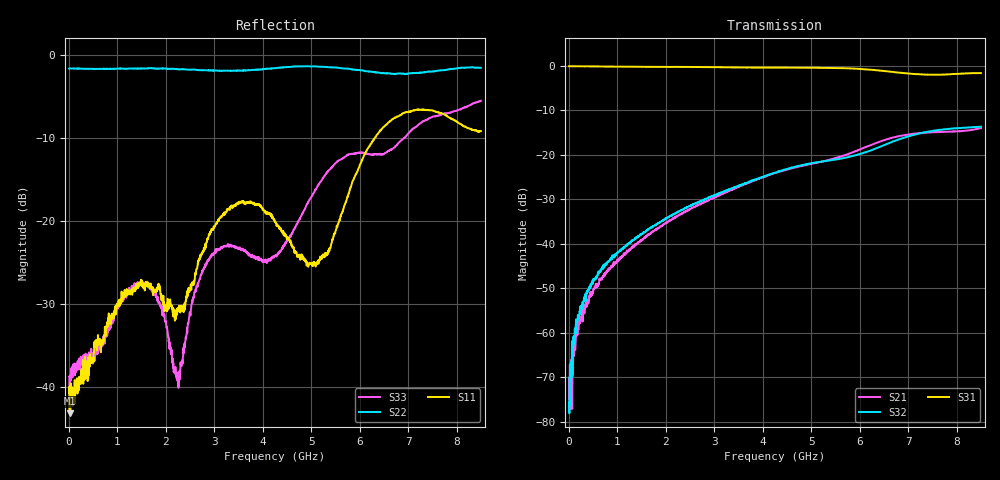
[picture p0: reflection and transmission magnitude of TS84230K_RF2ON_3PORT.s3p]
! Created with skrf (http://scikit-rf.org).
# Hz S RI R 50.0
!freq ReS11 ImS11 ReS12 ImS12 ReS13 ImS13
! ReS21 ImS21 ReS22 ImS22 ReS23 ImS23
! ReS31 ImS31 ReS32 ImS32 ReS33 ImS33
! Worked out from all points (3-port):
!   1601 points, 10 MHz to 8.5 GHz, reference 50 ohm
!   strongest paths, dB at 10 MHz, 2.132 GHz, 4.255 GHz, 6.378 GHz, 8.5 GHz:
!     S31: -0.1, -0.3, -0.4, -1.1, -1.7
!     S32: -75.6, -33.5, -24.0, -18.4, -13.7
!     S21: -70.3, -34.5, -24.1, -17.2, -14.0
!   lowest |S11| = -43.1 dB at 31.23 MHz (marker M1), VSWR 1.01, Z = 50.6 + j0.291 ohm
!   |S11| at or under -10 dB: start of sweep to 6.313 GHz
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1e7  0.0092 -0.00132  8.52e-05 -0.000126  0.987 -0.00469
     0.000144 0.00027  -0.8253 0.00436  -1.15e-05 0.000251
     0.9865 -0.0044  0.000139 9.03e-05  0.0116 0.000914
3.1225e7  0.00638 0.00287  7.66e-05 0.00025  0.9868 -0.00992
          -3.04e-05 0.000255  -0.8272 0.0111  0.000208 0.000189
          0.9864 -0.00997  0.000322 0.000303  0.0114 0.000235
2.275562e8  0.0102 0.00485  2.52e-05 0.00145  0.9824 -0.0667
            -4.62e-05 0.00128  -0.8209 0.0853  0.000177 0.00159
            0.982 -0.0667  0.00015 0.00176  0.0121 0.00433
8.749188e8  0.0184 0.0194  -0.00106 0.00553  0.9465 -0.2476
            -0.000712 0.00563  -0.7638 0.3048  -0.000136 0.00662
            0.9461 -0.2474  -6.77e-05 0.00699  0.00871 0.0229
1.628406e9  0.0293 0.031  -0.00317 0.012  0.8675 -0.4377
            -0.00318 0.0119  -0.6555 0.503  0.000342 0.0142
            0.8674 -0.4369  0.000111 0.0145  0.0138 0.04
2.254544e9  0.0262 -0.0118  -0.00458 0.0202  0.774 -0.5832
            -0.00462 0.0201  -0.5328 0.6187  0.00254 0.0224
            0.7749 -0.5822  0.00261 0.0227  -0.00632 0.00831
2.928438e9  -0.00976 -0.0866  -0.00426 0.0312  0.6429 -0.7186
            -0.00404 0.0315  -0.378 0.7082  0.00836 0.0327
            0.6428 -0.7176  0.00811 0.0327  -0.0602 -0.00885
4.255e9  -0.0154 -0.0987  0.011 0.0612  0.3252 -0.895
         0.0108 0.0615  0.06 0.828  0.0359 0.0518
         0.3264 -0.8944  0.0358 0.0518  -0.0608 0.0131
5.109306e9  0.00165 -0.0546  0.0322 0.0747  0.0787 -0.9451
            0.0318 0.075  0.2681 0.8071  0.0647 0.0507
            0.0803 -0.9442  0.0647 0.0508  -0.0809 0.1351
8.5e9  -0.316 0.1442  0.1989 0.0147  -0.6679 -0.4892
       0.1983 0.0156  0.8191 0.1598  0.1715 -0.1154
       -0.6645 -0.4911  0.1718 -0.115  0.1545 0.5053
